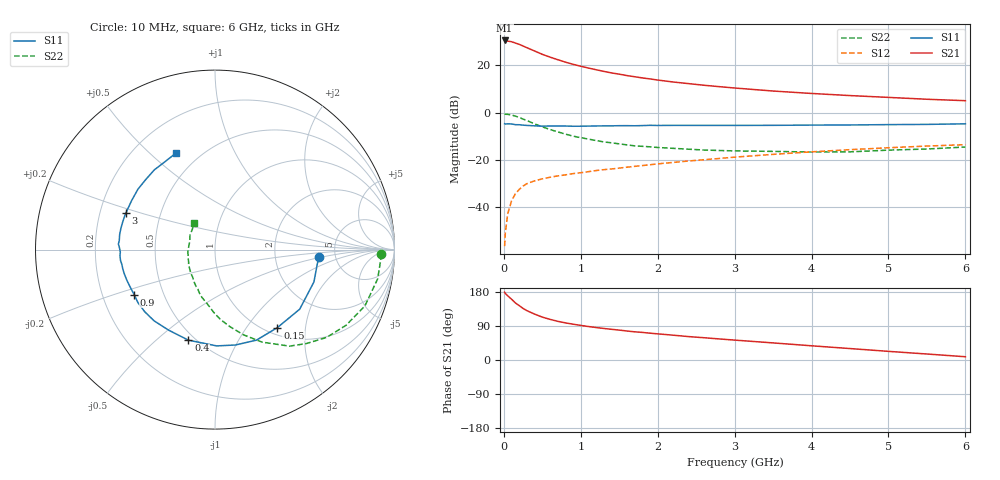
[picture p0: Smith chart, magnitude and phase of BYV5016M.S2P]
! SIEMENS Small Signal Semiconductors
! BFY420
! Si NPN RF SIEGET Grounded Emitter Transistor in MICRO-X
! VCE = 0.5 V  IC = 16 mA
! Common Emitter S-Parameters:  October  1996
# GHz  S  MA  R  50
!  f  S11  S21  S12  S22
! GHz  MAG  ANG  MAG  ANG  MAG  ANG  MAG  ANG
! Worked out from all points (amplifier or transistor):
!   36 points, 10 MHz to 6 GHz, reference 50 ohm
!   highest |S21| = 30.5 dB at 10 MHz (marker M1)
!   |S21| within 3 dB of that: start of sweep to 295.3 MHz
!   unconditionally stable (mu >= 1): 1.729 GHz to end of sweep
!   at 250 MHz: K = 0.29, MSG = 29.6 dB, |S12| = -31.1 dB
!   at 1.4 GHz: K = 0.92, MSG = 20.3 dB, |S12| = -23.8 dB
!   at 6 GHz: K = 1.13, MAG = 7.1 dB, |S12| = -13.5 dB
!   S11 on the Smith chart (normalised r, x): 10 MHz: 3.72, -0.49; 150 MHz: 1.12, -1.42; 400 MHz: 0.46, -0.64; 900 MHz: 0.34, -0.23; 3 GHz: 0.31, +0.18; 6 GHz: 0.37, +0.61
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0.01  0.5824 -4.3  33.62 178.8  0.0015 101.0  0.9258 -1.6
0.02  0.5757 -7.7  33.37 175.4  0.0029 80.6  0.9248 -3.8
0.05  0.5799 -18.1  32.58 169.5  0.0072 82.2  0.9208 -10.2
0.1  0.577 -35.1  31.62 160.4  0.0136 75.5  0.8922 -20.6
0.15  0.5565 -51.3  29.66 150.6  0.0193 68.7  0.8433 -30.0
0.2  0.5549 -65.4  27.81 143.5  0.0238 64.3  0.7912 -38.2
0.25  0.5435 -78.0  25.65 136.1  0.028 59.3  0.7301 -45.8
0.3  0.5366 -89.0  23.62 130.2  0.0315 56.9  0.6798 -52.3
0.4  0.5259 -106.4  20.12 121.1  0.0361 51.7  0.5787 -63.0
0.5  0.5179 -119.8  17.1 113.2  0.0398 48.9  0.5007 -71.5
0.6  0.5221 -130.5  14.94 107.3  0.043 46.9  0.4398 -78.7
0.7  0.5227 -138.5  13.2 102.1  0.0459 46.6  0.3925 -85.3
0.9  0.5155 -150.9  10.52 94.5  0.0514 45.8  0.3188 -95.6
1.1  0.5197 -160.6  8.776 88.3  0.0565 46.5  0.2759 -105.3
1.4  0.5254 -171.0  6.912 81.0  0.0644 46.5  0.2301 -117.4
1.6  0.5305 -176.3  6.076 76.5  0.0702 46.9  0.2083 -125.2
2.2  0.5378 171.1  4.45 65.5  0.0885 45.5  0.1759 -143.9
3  0.5367 157.7  3.321 52.5  0.1145 41.9  0.1551 -164.5
3.5  0.5389 149.5  2.864 45.1  0.1311 38.7  0.1515 -176.2
4.5  0.5488 134.7  2.296 30.2  0.1649 30.0  0.1481 161.4
5.5  0.5642 119.1  1.919 15.8  0.1964 20.0  0.1702 137.7
6  0.5804 111.9  1.79 8.6  0.2103 14.9  0.1876 128.5
